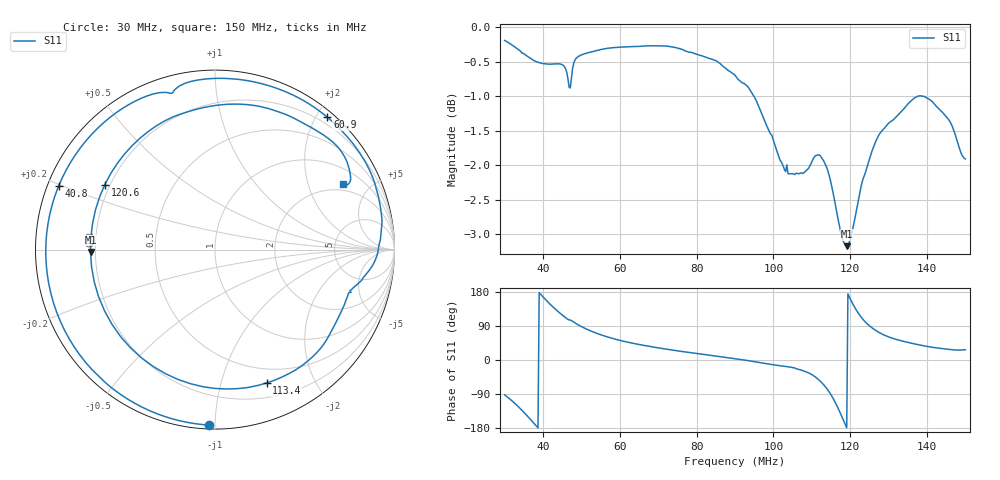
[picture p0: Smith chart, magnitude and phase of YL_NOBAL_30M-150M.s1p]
!File
# Hz S RI R 50
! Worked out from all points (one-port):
!   401 points, 30 MHz to 150 MHz, reference 50 ohm
!   lowest |S11| = -3.2 dB at 119.1 MHz (marker M1), VSWR 5.53, Z = 9.04 - j0.459 ohm
!   |S11| at or under -10 dB: nowhere
!   S11 on the Smith chart (normalised r, x): 30 MHz: 0.02, -0.97; 40.8 MHz: 0.03, +0.19; 60.9 MHz: 0.09, +2.16; 113.4 MHz: 0.34, -1.40; 120.6 MHz: 0.18, +0.26; 150 MHz: 1.66, +3.40
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3e7  -0.0341 -0.9775
3.33e7  -0.4893 -0.8314
3.66e7  -0.8629 -0.3964
3.87e7  -0.943 -0.0154
4.08e7  -0.8718 0.3528
4.29e7  -0.6882 0.6408
4.5e7  -0.4515 0.8237
4.89e7  -0.0721 0.9481
5.25e7  0.2266 0.9322
6e7  0.5971 0.7609
6.09e7  0.626 0.7376
7.5e7  0.8808 0.3961
9e7  0.9214 0.0545
1.05e8  0.7359 -0.2671
1.104e8  0.6058 -0.5274
1.134e8  0.2869 -0.7432
1.149e8  -0.00208 -0.7733
1.161e8  -0.2756 -0.6915
1.176e8  -0.5744 -0.4156
1.191e8  -0.6936 -0.0132
1.2e8  -0.6656 0.2226
1.206e8  -0.6139 0.3619
1.227e8  -0.3253 0.6904
1.248e8  -0.0291 0.798
1.29e8  0.3552 0.7671
1.35e8  0.6052 0.6383
1.416e8  0.7379 0.4825
1.5e8  0.7145 0.3654
